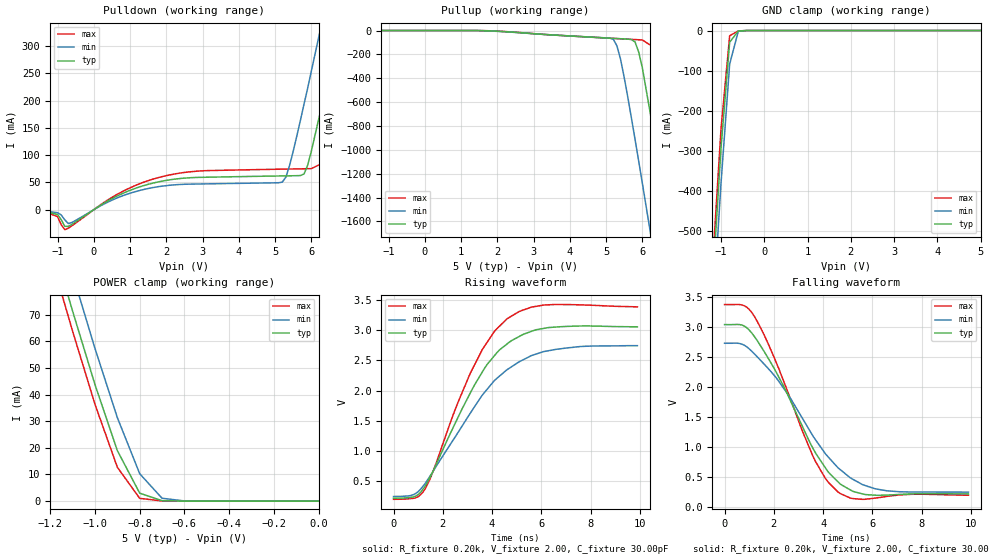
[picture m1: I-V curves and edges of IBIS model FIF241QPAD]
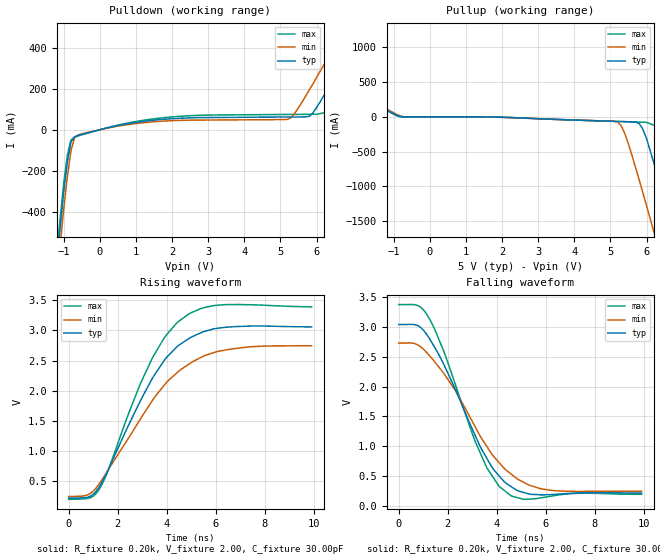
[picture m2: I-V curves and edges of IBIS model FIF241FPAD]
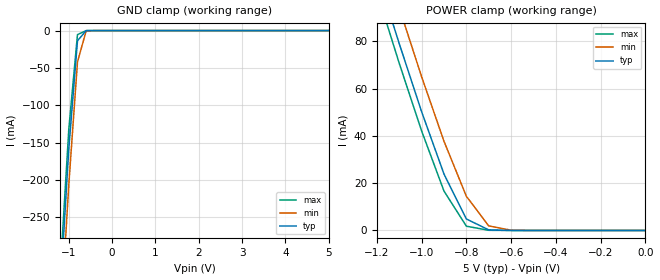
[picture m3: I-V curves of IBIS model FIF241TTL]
| IBIS file idt72831.ibs created by s2ibis2 version 1.1
| North Carolina State University Electronics Research Laboratory  1995
[IBIS ver]   2.1
[File name]   idt72831.ibs
[File Rev]   1.0
[Date]   08/22/97
[Source]   Integrated Device Technology, Inc.
[Notes]   1. Temperatures: typ=25C, min=70C, max=0C 2. Cemos8_5v
   process. 3. Ramp rates based on 50 ohm load.
[Copyright]   Copyright 1997, Integrated Device Technology, Inc.
|   Component idt72831
[Component]   idt72831
[Manufacturer]   Integrated Device Technology
[Package]
| variable   typ   min   max
R_pkg   0.75   0.60   0.90
L_pkg   8.10nH   8.30nH   9.90nH
C_pkg   0.53pF   0.46pF   0.60pF
[Pin]  signal_name   model_name   R_pin   L_pin   C_pin
1   QA1   FIF241QPAD
2   QA2   FIF241QPAD
3   QA3   FIF241QPAD
4   QA4   FIF241QPAD
5   QA5   FIF241QPAD
6   QA6   FIF241QPAD
7   QA7   FIF241QPAD
8   QA8   FIF241QPAD
9   VCC   POWER
10   WENA2   FIF241TTL
11   WCLKA   FIF241TTL
12   WENAL1   FIF241TTL
13   RSAL   FIF241TTL
14   DA8   FIF241TTL
15   DA7   FIF241TTL
16   DA6   FIF241TTL
17   DA5   FIF241TTL
18   DA4   FIF241TTL
19   DA3   FIF241TTL
20   DA2   FIF241TTL
21   DA1   FIF241TTL
22   DA0   FIF241TTL
23   PAFAL   FIF241FPAD
24   PAEAL   FIF241FPAD
25   WENB2   FIF241TTL
26   WCLKB   FIF241TTL
27   WENBL1   FIF241TTL
28   RSBL   FIF241TTL
29   DB8   FIF241TTL
30   DB7   FIF241TTL
31   DB6   FIF241TTL
32   DB5   FIF241TTL
33   DB4   FIF241TTL
34   DB3   FIF241TTL
35   DB2   FIF241TTL
36   DB1   FIF241TTL
37   DB0   FIF241TTL
38   PAFBL   FIF241FPAD
39   PAEBL   FIF241FPAD
40   VCC   POWER
41   GND   GND
42   RENBL1   FIF241TTL
43   RCLKB   FIF241TTL
44   RENBL2   FIF241TTL
45   OEBL   FIF241TTL
46   EFBL   FIF241FPAD
47   FFBL   FIF241FPAD
48   QB0   FIF241QPAD
49   QB1   FIF241QPAD
50   QB2   FIF241QPAD
51   QB3   FIF241QPAD
52   QB4   FIF241QPAD
53   QB5   FIF241QPAD
54   QB6   FIF241QPAD
55   QB7   FIF241QPAD
56   QB8   FIF241QPAD
57   GND   GND
58   RENAL1   FIF241TTL
59   RCLKA   FIF241TTL
60   RENAL2   FIF241TTL
61   OEAL   FIF241TTL
62   EFAL   FIF241FPAD
63   FFAL   FIF241FPAD
64   QA0   FIF241QPAD
| Models and submodels in the file (3): FIF241QPAD (3-state), FIF241FPAD (Output), FIF241TTL (Input)
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| FIN  FIN   dummy_model
| QIN  QIN   dummy_model
| QOEL QOEL   dummy_model
|   Model FIF241QPAD
[Model]   FIF241QPAD
Model_type   3-state
Polarity   Non-Inverting
Enable   Active-Low
Vmeas =  1.500V
C_comp   3.00pF   NA   NA
[Temperature Range]   25.00   70.00   0.000
[Voltage Range]   5.00V   4.50V   5.50V
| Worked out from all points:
|   slope of the pulldown table from 0 to 0.75 V, typ, clamps not added: 26.4 ohm
|   GND clamp passes 1 mA (typ) near -0.58 V on its own axis
|   POWER clamp passes 1 mA (typ) near -0.73 V on its own axis
|   rising waveform, R_fixture 0.20k, V_fixture 2.00, C_fixture 30.00pF: 20-80 % time 2.17ns typ, 2.59ns min, 1.95ns max; typ from 0.212 V to 3.06 V
|   falling waveform, R_fixture 0.20k, V_fixture 2.00, C_fixture 30.00pF: 20-80 % time 2.11ns typ, 2.47ns min, 1.85ns max; typ from 3.04 V to 0.213 V
[Pulldown]
| voltage   I(typ)   I(min)   I(max)
-5V       0A         0A         0A
-1.4V     -3mA       -2mA       -2.6mA
-800mV    -30.42mA   -18.6mA    -36.69mA
1.7V      49.86mA    41.4mA     57.4mA
5.2V      62.01mA    50.61mA    74.43mA
5.4V      62.22mA    81.07mA    74.66mA
5.8V      65.63mA    194mA      75.11mA
6V        107mA      254mA      75.33mA
6.4V      223mA      376mA      88.46mA
6.8V      345mA      500mA      198mA
7.2V      469mA      624mA      320mA
10V       1.346A     1.502A     1.195A
[Pullup]
| voltage   I(typ)   I(min)   I(max)
-5V       0A         0A         0A
1.5V      -479uA     -1.046mA   -164uA
5.2V      -65.7mA    -73.36mA   -65.97mA
5.3V      -67.33mA   -129mA     -67.59mA
5.4V      -68.96mA   -242mA     -69.22mA
5.8V      -96.18mA   -914mA     -75.69mA
6V        -312mA     -1.279A    -78.93mA
6.4V      -1.008A    -2.023A    -157mA
6.8V      -1.75A     -2.776A    -778mA
7.2V      -2.503A    -3.534A    -1.516A
7.6V      -3.262A    -4.295A    -2.268A
10V       -7.849A    -8.885A    -6.849A
[GND_clamp]
| voltage   I(typ)   I(min)   I(max)
-5V       -7.849A    -7.926A    -7.807A
-1.2V     -640mA     -729mA     -591mA
-1V       -293mA     -381mA     -246mA
-800mV    -29.29mA   -83.51mA   -12.91mA
-600mV    -1.086mA   -1.828mA   -995uA
-400mV    -11.7nA    -1.657uA   -4.457nA
5V        50nA       1.239uA    50nA
[POWER_clamp]
| voltage   I(typ)   I(min)   I(max)
-5V       1.28A      1.292A     1.273A
-1.2V     100mA      114mA      92.56mA
-1.1V     71.31mA    85.16mA    63.76mA
-1V       43.75mA    57.31mA    36.34mA
-900mV    18.98mA    31.36mA    12.72mA
-800mV    2.991mA    10.3mA     1.049mA
-700mV    169uA      1.084mA    64.47uA
-600mV    6.517uA    77.91uA    260nA
0V        50nA       45nA       55nA
[Ramp]
| variable   typ   min   max
dV/dt_r   1.00/1.23n   0.85/1.56n   1.15/1.10n
dV/dt_f   1.67/2.34n   1.36/2.85n   1.96/2.01n
R_load = 50.00
[Rising Waveform]
R_fixture = 0.20k
V_fixture = 2.00
C_fixture = 30.00pF
R_dut = 0.75
L_dut = 8.10nH
C_dut = 0.53pF
| time   V(typ)   V(min)   V(max)
0s        212mV      240mV      193mV
900ps     246mV      290mV      218mV
1.3ns     421mV      464mV      378mV
3.1ns     1.947V     1.614V     2.272V
3.8ns     2.434V     2.021V     2.802V
4.6ns     2.771V     2.344V     3.19V
5.3ns     2.94V      2.52V      3.343V
6.1ns     3.033V     2.648V     3.421V
7.6ns     3.073V     2.732V     3.424V
9.9ns     3.059V     2.746V     3.391V
[Falling Waveform]
R_fixture = 0.20k
V_fixture = 2.00
C_fixture = 30.00pF
R_dut = 0.75
L_dut = 8.10nH
C_dut = 0.53pF
| time   V(typ)   V(min)   V(max)
0s        3.045V     2.733V     3.38V
800ps     3.021V     2.7V       3.36V
1.2ns     2.852V     2.56V      3.19V
2.2ns     2.168V     2.097V     2.31V
3.6ns     967mV      1.174V     833mV
4.1ns     647mV      881mV      468mV
4.6ns     419mV      653mV      248mV
5.2ns     258mV      460mV      136mV
6.2ns     190mV      293mV      148mV
9.9ns     213mV      243mV      192mV
|   Model FIF241FPAD
[Model]   FIF241FPAD
Model_type   Output
Vmeas =  1.500V
C_comp   3.00pF   NA   NA
[Temperature Range]   25.00   70.00   0.000
[Voltage Range]   5.00V   4.50V   5.50V
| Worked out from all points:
|   slope of the pulldown table from 0 to 0.75 V, typ, clamps not added: 26.4 ohm
|   rising waveform, R_fixture 0.20k, V_fixture 2.00, C_fixture 30.00pF: 20-80 % time 2.15ns typ, 2.57ns min, 1.96ns max; typ from 0.212 V to 3.06 V
|   falling waveform, R_fixture 0.20k, V_fixture 2.00, C_fixture 30.00pF: 20-80 % time 1.91ns typ, 2.24ns min, 1.69ns max; typ from 3.04 V to 0.212 V
[Pulldown]
| voltage   I(typ)   I(min)   I(max)
-5V       -7.849A    -7.926A    -7.807A
-1.4V     -1.006A    -1.093A    -958mA
-1V       -302mA     -386mA     -259mA
-800mV    -59.72mA   -102mA     -49.6mA
-600mV    -27.75mA   -25.16mA   -30.34mA
5.2V      62.01mA    50.61mA    74.43mA
5.8V      65.63mA    194mA      75.11mA
6.4V      223mA      376mA      88.46mA
6.8V      345mA      500mA      198mA
7.2V      469mA      624mA      320mA
8V        718mA      874mA      568mA
10V       1.346A     1.502A     1.195A
[Pullup]
| voltage   I(typ)   I(min)   I(max)
-5V       1.28A      1.292A     1.273A
-1.4V     160mA      173mA      152mA
-800mV    2.991mA    10.3mA     1.049mA
5.2V      -65.7mA    -73.36mA   -65.97mA
5.4V      -68.96mA   -242mA     -69.22mA
5.8V      -96.18mA   -914mA     -75.69mA
6V        -312mA     -1.279A    -78.93mA
6.4V      -1.008A    -2.023A    -157mA
6.8V      -1.75A     -2.776A    -778mA
7.2V      -2.503A    -3.534A    -1.516A
7.6V      -3.262A    -4.295A    -2.268A
10V       -7.849A    -8.885A    -6.849A
[Ramp]
| variable   typ   min   max
dV/dt_r   1.00/1.24n   0.85/1.51n   1.15/1.07n
dV/dt_f   1.67/1.85n   1.36/2.26n   1.96/1.61n
R_load = 50.00
[Rising Waveform]
R_fixture = 0.20k
V_fixture = 2.00
C_fixture = 30.00pF
R_dut = 0.75
L_dut = 8.10nH
C_dut = 0.53pF
| time   V(typ)   V(min)   V(max)
0s        212mV      240mV      193mV
800ps     231mV      272mV      210mV
1.3ns     435mV      482mV      396mV
2.9ns     1.812V     1.512V     2.092V
3.4ns     2.196V     1.827V     2.533V
3.9ns     2.506V     2.092V     2.88V
4.5ns     2.757V     2.327V     3.156V
5.4ns     2.964V     2.553V     3.365V
6.1ns     3.037V     2.653V     3.42V
9.9ns     3.058V     2.745V     3.391V
[Falling Waveform]
R_fixture = 0.20k
V_fixture = 2.00
C_fixture = 30.00pF
R_dut = 0.75
L_dut = 8.10nH
C_dut = 0.53pF
| time   V(typ)   V(min)   V(max)
0s        3.045V     2.733V     3.38V
800ps     3.022V     2.698V     3.36V
1.2ns     2.843V     2.547V     3.178V
1.8ns     2.406V     2.246V     2.634V
2.3ns     1.963V     1.942V     2.048V
3.1ns     1.197V     1.339V     1.097V
3.6ns     791mV      991mV      631mV
4.5ns     343mV      558mV      192mV
6ns       184mV      271mV      146mV
9.9ns     212mV      242mV      191mV
|   Model FIF241TTL
[Model]   FIF241TTL
Model_type   Input
Vinl =  0.000V
Vinh =  3.000V
Vmeas =  1.500V
C_comp   3.00pF   NA   NA
[Temperature Range]   25.00   70.00   0.000
[Voltage Range]   5.00V   4.50V   5.50V
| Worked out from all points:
|   GND clamp passes 1 mA (typ) near -0.61 V on its own axis
|   POWER clamp passes 1 mA (typ) near -0.72 V on its own axis
[GND_clamp]
| voltage   I(typ)   I(min)   I(max)
-5V       -4.391A    -4.433A    -4.368A
-1.2V     -352mA     -401mA     -325mA
-1V       -158mA     -206mA     -132mA
-800mV    -13.65mA   -42.02mA   -5.426mA
-600mV    -95.68uA   -488uA     -19.8uA
5V        50nA       2.529uA    50nA
[POWER_clamp]
| voltage   I(typ)   I(min)   I(max)
-5V       1.33A      1.343A     1.323A
-1.2V     109mA      124mA      101mA
-1.1V     79.07mA    94.22mA    70.74mA
-1V       50.25mA    65.05mA    42.12mA
-900mV    23.87mA    37.74mA    16.67mA
-800mV    4.863mA    14.45mA    1.814mA
-700mV    253uA      1.929mA    79.02uA
-600mV    7.842uA    115uA      476nA
0V        50nA       45nA       55nA
